(* Logix 5000 AddOnInstructionDefinition export RTA_435NBX_490NBX_Gateway_to_PLC; software revision 20.01 *)

TYPE RTA_STRING_4096 :   // string type; String Data Type with up to 4096 characters available
STRUCT
   LEN : DINT;
   DATA : SINT[4096];
END_STRUCT
END_TYPE

ADD_ON_INSTRUCTION RTA_435NBX_490NBX_Gateway_to_PLC   (* revision 1.0, vendor Real Time Automation, Inc. *)
// RTA's 435NBX / 490NBX Gateway to PLC handshaking
VAR_IN_OUT
   DataIn : RTA_STRING_4096; {required}
   DataOut : RTA_STRING_4096; {required}
END_VAR
VAR
   DataFromGateway : RTA_STRING_4096; {access None}
   DataToCustomer : RTA_STRING_4096; {access None}
END_VAR

ROUTINE Logic   (* ladder *)
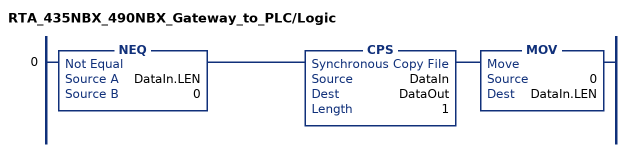
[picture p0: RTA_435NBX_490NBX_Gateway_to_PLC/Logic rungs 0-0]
   0: NEQ(DataIn.LEN,0)CPS(DataIn,DataOut,1)MOV(0,DataIn.LEN);
END_ROUTINE
END_ADD_ON_INSTRUCTION
